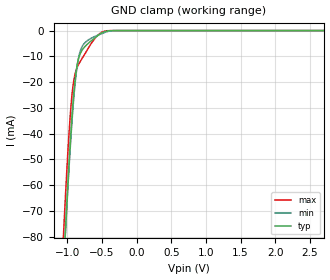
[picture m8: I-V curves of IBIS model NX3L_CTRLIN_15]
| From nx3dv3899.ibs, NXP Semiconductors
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|   Model NX3L_CTRLIN_15
[Model]   NX3L_CTRLIN_15
Model_type   Input
Vinl = 0.5250V
Vinh = 0.9750V
C_comp   0.76pF   0.60pF   0.99pF
[Model Spec]
| Note: The input and output voltage ratings may be exceeded if the input and
|   output current ratings are observed (please refer to the data sheet)
|   Subparameter   typ   min   max
| Thresholds
Vinh   0.9750   0.9100   1.0400
Vinl   0.5250   0.4900   0.5600
| Overshoot
S_overshoot_high   3.6   3.6   3.6
S_overshoot_low   -0.5   -0.5   -0.5
D_overshoot_high   5.4   5.4   5.4
D_overshoot_low   -0.95   -0.9   -1.0
D_overshoot_time   3n   3n   3n
|Ambient temperature:   25   85   -40
[Temperature Range]   30   90   -35
[Voltage Range]   1.5   1.4   1.6
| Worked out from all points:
|   GND clamp passes 1 mA (typ) near -0.51 V on its own axis
|Process Range   nominal   slow   fast
[GND_clamp]
|   voltage   I(typ)   I(min)   I(max)
-4.3V     -2.211A    -2.201A    -2.207A
-1.065V   -97.92mA   -98.07mA   -84.2mA
-1.05V    -89.65mA   -90.03mA   -75.98mA
-1.035V   -81.53mA   -82.14mA   -67.97mA
-1.02V    -73.59mA   -74.44mA   -60.23mA
-975mV    -51.22mA   -52.7mA    -39.27mA
-930mV    -32.11mA   -33.91mA   -24mA
-885mV    -18.31mA   -19.54mA   -16.43mA
-840mV    -11mA      -10.77mA   -13.24mA
-750mV    -6.311mA   -4.808mA   -9.171mA
-480mV    -607.1uA   -962.6uA   -390.3uA
4.3V      0A         0A         0A
